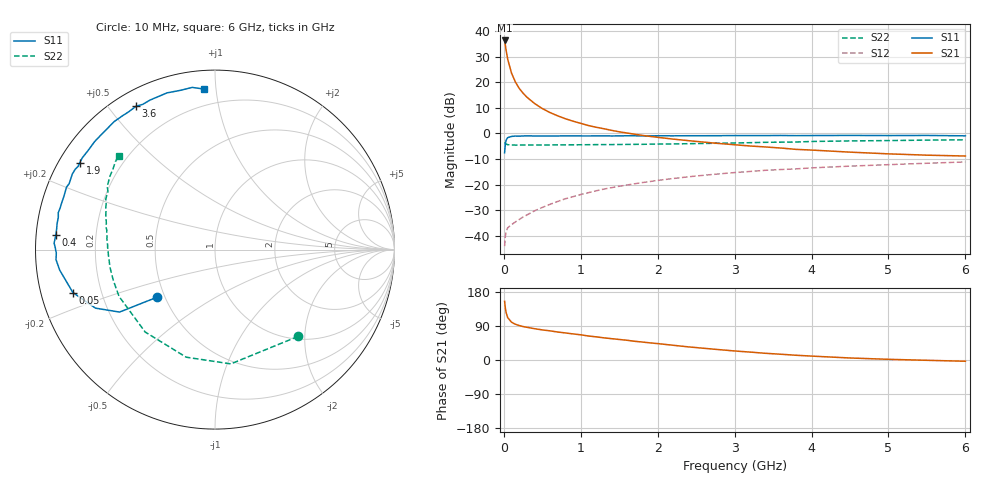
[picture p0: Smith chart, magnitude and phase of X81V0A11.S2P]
! SIEMENS Small Signal Semiconductors
! BFP136W
! Si NPN RF Bipolar Junction Transistor in SOT343
! VCE = 1 V  IC = 110 mA
! Common Emitter S-Parameters:  September  1994
# GHz  S  MA  R  50
!  f  S11  S21  S12  S22
! GHz  MAG  ANG  MAG  ANG  MAG  ANG  MAG  ANG
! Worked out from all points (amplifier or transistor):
!   40 points, 10 MHz to 6 GHz, reference 50 ohm
!   highest |S21| = 36.3 dB at 10 MHz (marker M1)
!   |S21| within 3 dB of that: start of sweep to 25.48 MHz
!   unconditionally stable (mu >= 1): 382.2 MHz to 3.522 GHz; 3.634 GHz to 4.196 GHz; 4.695 GHz to 5.338 GHz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
!   at 200 MHz: K = 0.80, MSG = 25.6 dB, |S12| = -33.6 dB
!   at 1.5 GHz: K = 1.14, MAG = 8.3 dB, |S12| = -20.6 dB
!   at 6 GHz: K = 1.04, MAG = 0.0 dB, |S12| = -11.1 dB
!   S11 on the Smith chart (normalised r, x): 10 MHz: 0.45, -0.29; 50 MHz: 0.10, -0.15; 400 MHz: 0.06, +0.05; 1.9 GHz: 0.06, +0.29; 3.6 GHz: 0.06, +0.59; 6 GHz: 0.10, +0.93
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0.01  0.4181 -140.6  65.16 154.9  0.0063 61.2  0.6692 -46.3
0.02  0.6356 -146.8  52.36 136.2  0.01 49.8  0.6428 -82.1
0.03  0.7415 -153.9  41.55 124.6  0.0122 41.8  0.6206 -105.0
0.05  0.8271 -163.2  28.11 111.9  0.0144 34.0  0.6018 -130.3
0.1  0.873 -172.5  15 99.7  0.0166 34.7  0.5948 -154.0
0.15  0.8875 -176.4  10.1 94.3  0.0187 38.9  0.5919 -162.9
0.2  0.8843 -178.8  7.557 90.9  0.0209 43.6  0.5919 -167.5
0.25  0.8912 179.0  6.09 88.2  0.0234 46.9  0.5935 -170.6
0.3  0.8972 177.7  5.088 86.3  0.0256 50.4  0.5927 -172.6
0.4  0.8904 174.7  3.829 82.6  0.0309 54.9  0.594 -175.5
0.5  0.8897 172.4  3.055 79.4  0.0359 57.7  0.5949 -177.5
0.7  0.8914 168.3  2.201 73.8  0.047 61.6  0.5972 179.9
0.9  0.8934 165.1  1.732 68.8  0.0582 62.3  0.5988 177.6
1.1  0.8925 160.6  1.424 63.3  0.0698 62.4  0.6019 175.9
1.5  0.8945 154.2  1.074 54.2  0.0931 60.9  0.6074 172.5
1.9  0.8952 147.2  0.875 45.2  0.1151 57.7  0.6164 169.1
2.2  0.8971 141.9  0.774 38.9  0.1316 54.9  0.6229 166.4
3.2  0.9063 124.9  0.568 20.9  0.1808 44.4  0.6586 157.0
3.6  0.9117 118.8  0.518 15.2  0.1971 40.2  0.6744 153.4
4.5  0.9132 107.0  0.431 5.3  0.2298 31.4  0.7136 145.2
5.5  0.9126 98.0  0.376 -0.8  0.2616 23.4  0.74 138.6
6  0.8964 93.9  0.362 -3.3  0.2774 19.0  0.75 135.7
